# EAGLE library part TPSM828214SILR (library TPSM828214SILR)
Switching Voltage Regulators 5.5-V input, 1-A step-down module with integrated inductor in 2 x 2.5 x 1.1-mm SIP package Source: Datasheet
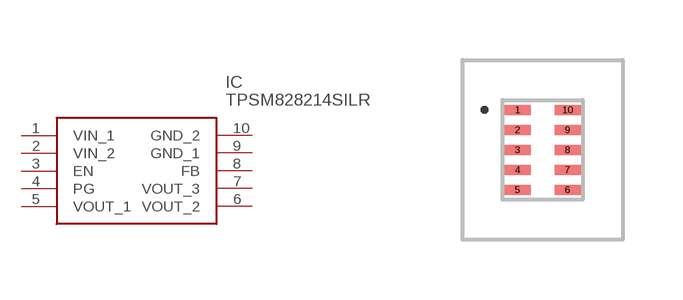
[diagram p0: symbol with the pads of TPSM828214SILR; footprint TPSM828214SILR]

Designator prefix IC

## TPSM828214SILR (Arrow_Part_Number: TPSM828214SILR; Arrow_Price-Stock: https://www.arrow.com/en/products/tpsm828214silr/texas-instruments?region=nac; Description: Switching Voltage Regulators 5.5-V input, 1-A step-down module with integrated inductor in 2 x 2.5 x 1.1-mm SIP package; Height: 1.1mm; Manufacturer_Name: Texas Instruments; Manufacturer_Part_Number: TPSM828214SILR; Mouser_Part_Number: 595-TPSM828214SILR; Mouser_Price-Stock: https://www.mouser.co.uk/ProductDetail/Texas-Instruments/TPSM828214SILR?qs=iLbezkQI%252BsibRGaNc1MtTA%3D%3D)  [TPSM828214SILR]
1  VIN_1
2  VIN_2
3  EN
4  PG
5  VOUT_1
6  VOUT_2
7  VOUT_3
8  FB
9  GND_1
10  GND_2

## Footprint TPSM828214SILR (pad centres in mm)
SIL0010D_2021
smd 0.65 x 0.25: 1 -0.625,1; 2 -0.625,0.5; 3 -0.625,0; 4 -0.625,-0.5; 5 -0.625,-1; 6 0.625,-1; 7 0.625,-0.5; 8 0.625,0; 9 0.625,0.5; 10 0.625,1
